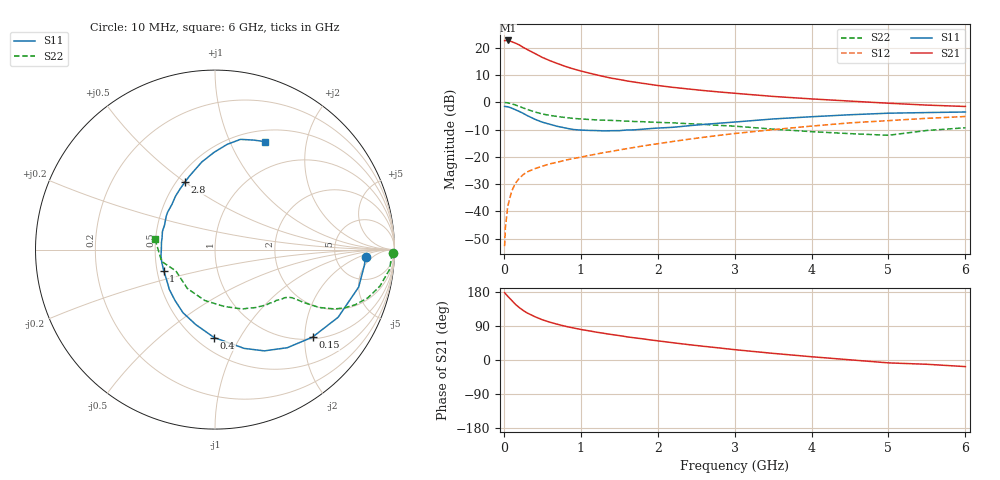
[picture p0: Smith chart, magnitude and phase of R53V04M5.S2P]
! SIEMENS Small Signal Semiconductors
! BFR183
! Si NPN RF Bipolar Junction Transistor in SOT23
! VCE = 3 V  IC = 4.5 mA
! Common Emitter S-Parameters:  May  1996
# GHz  S  MA  R  50
!  f  S11  S21  S12  S22
! GHz  MAG  ANG  MAG  ANG  MAG  ANG  MAG  ANG
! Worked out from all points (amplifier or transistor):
!   36 points, 10 MHz to 6 GHz, reference 50 ohm
!   highest |S21| = 22.7 dB at 50 MHz (marker M1)
!   |S21| within 3 dB of that: start of sweep to 282.6 MHz
!   unconditionally stable (mu >= 1): 1.082 GHz to 2.658 GHz
!   at 250 MHz: K = 0.39, MSG = 23.4 dB, |S12| = -26.6 dB
!   at 1.4 GHz: K = 1.06, MAG = 11.9 dB, |S12| = -18.0 dB
!   at 6 GHz: K = 0.89, MSG = 1.8 dB, |S12| = -5.2 dB
!   S11 on the Smith chart (normalised r, x): 10 MHz: 11, -3; 150 MHz: 1.05, -2.19; 400 MHz: 0.61, -0.78; 1 GHz: 0.54, -0.14; 2.8 GHz: 0.55, +0.50; 6 GHz: 0.64, +1.36
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0.01  0.8399 -2.9  13.51 177.9  0.0023 89.5  0.9913 -1.2
0.02  0.8366 -6.1  13.53 175.2  0.005 83.8  0.984 -2.6
0.05  0.8273 -14.6  13.59 168.4  0.0122 83.4  0.9783 -6.6
0.1  0.7828 -28.8  12.95 157.8  0.0231 75.5  0.9411 -12.5
0.15  0.73 -41.9  12.14 147.0  0.0327 69.8  0.8931 -17.5
0.2  0.6791 -53.6  11.26 138.5  0.0403 65.0  0.8392 -21.5
0.25  0.6277 -64.0  10.19 131.0  0.0469 61.0  0.7879 -24.4
0.3  0.5742 -73.5  9.326 124.5  0.0526 58.7  0.7433 -26.4
0.4  0.4899 -90.6  7.886 114.6  0.0605 55.5  0.6654 -29.0
0.5  0.4314 -104.4  6.649 106.2  0.0673 54.3  0.6099 -30.1
0.6  0.3943 -116.9  5.779 99.7  0.0743 53.9  0.5739 -30.8
0.8  0.3377 -138.9  4.547 89.0  0.0867 54.4  0.5253 -31.6
1  0.309 -157.6  3.747 80.7  0.0985 55.9  0.4945 -32.6
1.1  0.3049 -166.3  3.452 77.2  0.1054 56.5  0.4844 -33.5
1.3  0.2989 179.5  2.96 70.4  0.1195 57.0  0.4695 -35.0
1.6  0.31 160.8  2.461 61.2  0.1413 57.7  0.4506 -38.5
2.2  0.3478 133.6  1.876 45.5  0.1914 56.7  0.4193 -47.5
2.8  0.4132 113.6  1.545 31.8  0.2475 52.8  0.3767 -59.9
3.5  0.4941 98.5  1.28 17.5  0.3148 45.9  0.3214 -80.6
4.5  0.5902 83.4  1.051 0.5  0.4192 34.0  0.266 -125.3
5.5  0.6473 70.5  0.887 -11.3  0.5078 21.3  0.3043 -167.4
6  0.663 65.1  0.837 -17.4  0.5483 13.0  0.3407 169.6
